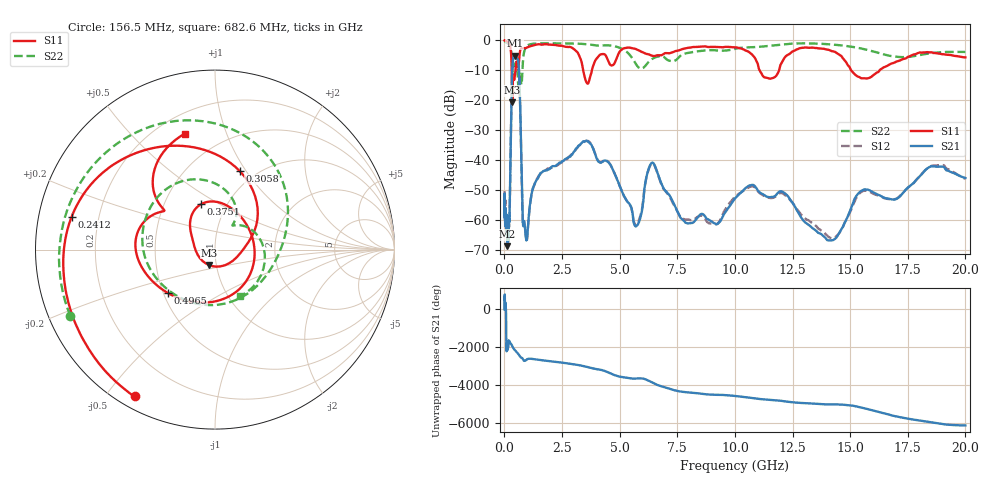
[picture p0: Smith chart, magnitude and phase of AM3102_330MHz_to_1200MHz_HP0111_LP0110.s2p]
! Date/Time: Tue, Sep 11, 2018 5:16 PM
! Network Analyzer: Agilent Technologies E8362B Rev: A.07.50.63
! Sweep from 0.010 to 20.000 GHz, 1601 Points, Sweep Type: LOG
! Power Supply: 4.949 V, 0.001 A
# Hz S DB R 50
!freq MagS11 AngS11 MagS21 AngS21 MagS12 AngS12 MagS22 AngS22
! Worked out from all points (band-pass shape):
!   1601 points, 10 MHz to 20 GHz, reference 50 ohm
!   highest |S21| = -5.05 dB at 447.2 MHz (marker M1); lowest = -68.7 dB at 121.7 MHz (marker M2)
!   |S21| within 3 dB of the highest: 352.4 MHz to 615.5 MHz (263.1 MHz wide, 54.4 % of centre)
!   lowest |S11| = -20.7 dB at 341.1 MHz (marker M3), VSWR 1.20, Z = 46 - j7.98 ohm
!   |S11| at or under -10 dB: 3.418 GHz to 3.797 GHz (379.5 MHz wide, 10.5 % of centre); 11.07 GHz to 11.92 GHz (844.2 MHz wide, 7.34 % of centre); 15.04 GHz to 16.28 GHz (1.236 GHz wide, 7.89 % of centre)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
!   |S22| runs from -15.6 to -0.2 dB; largest |S21 - S12| = 0.0097
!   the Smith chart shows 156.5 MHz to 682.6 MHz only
!   S11 on the Smith chart (normalised r, x): 156.5 MHz: 0.05, -0.59; 241.2 MHz: 0.10, +0.11; 305.8 MHz: 0.84, +0.94; 375.1 MHz: 0.76, +0.41; 496.5 MHz: 0.53, -0.29; 682.6 MHz: 0.31, +0.73
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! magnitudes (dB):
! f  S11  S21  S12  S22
! 10 MHz  0.0  -54.1  -53.3  -0.2
! 35.55 MHz  0.0  -61.3  -59.0  -0.4
! 121.7 MHz  -0.4  -68.7  -64.9  -0.9
! 126.4 MHz  -0.4  -65.7  -64.6  -0.9
! 156.5 MHz  -0.6  -64.2  -66.9  -1.0
! 241.2 MHz  -1.7  -52.2  -52.2  -1.8
! 305.8 MHz  -6.8  -20.5  -20.5  -4.0
! 341.1 MHz  -20.7  -9.6  -9.7  -8.3
! 375.1 MHz  -11.6  -6.4  -6.5  -10.3
! 447.2 MHz  -12.2  -5.0  -5.1  -8.2
! 496.5 MHz  -9.0  -5.3  -5.4  -7.3
! 682.6 MHz  -3.5  -21.1  -21.2  -10.6
! 794.6 MHz  -2.7  -59.8  -60.0  -8.3
! 938.4 MHz  -2.5  -66.2  -66.0  -2.2
! 1.59 GHz  -1.4  -44.2  -44.3  -1.0
! 3.617 GHz  -14.4  -33.7  -33.5  -1.3
! 5.652 GHz  -2.8  -61.7  -61.2  -7.2
! 6.426 GHz  -5.2  -40.8  -41.1  -6.1
! 7.882 GHz  -2.6  -60.9  -59.8  -4.3
! 10.73 GHz  -4.6  -48.2  -48.7  -2.3
! 14.07 GHz  -3.1  -66.8  -65.6  -1.3
! 20 GHz  -5.7  -45.9  -46.2  -3.9
